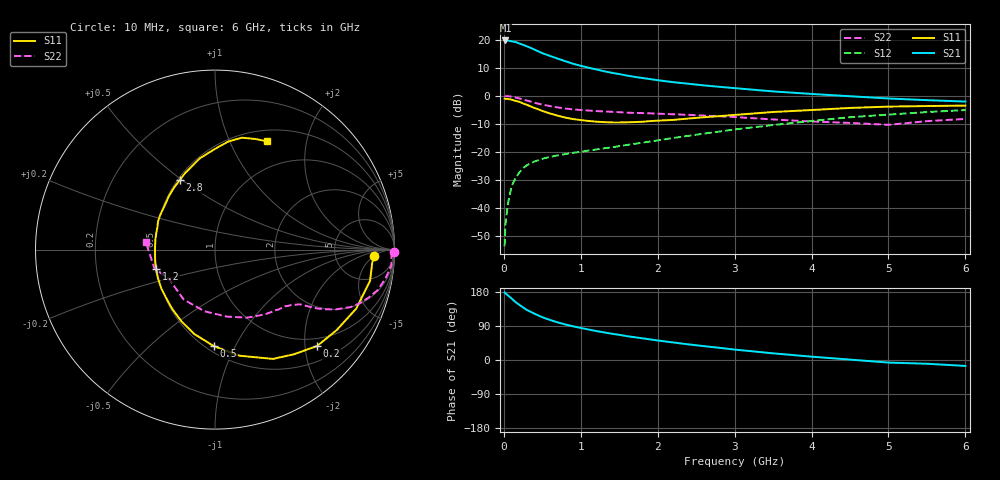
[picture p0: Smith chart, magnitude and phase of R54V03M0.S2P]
! SIEMENS Small Signal Semiconductors
! BFR183
! Si NPN RF Bipolar Junction Transistor in SOT23
! VCE = 4 V  IC = 3 mA
! Common Emitter S-Parameters:  May  1996
# GHz  S  MA  R  50
!  f  S11  S21  S12  S22
! GHz  MAG  ANG  MAG  ANG  MAG  ANG  MAG  ANG
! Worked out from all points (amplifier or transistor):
!   36 points, 10 MHz to 6 GHz, reference 50 ohm
!   highest |S21| = 19.7 dB at 20 MHz (marker M1)
!   |S21| within 3 dB of that: start of sweep to 377.3 MHz
!   unconditionally stable (mu >= 1): 1.261 GHz to 2.751 GHz
!   at 250 MHz: K = 0.29, MSG = 22.0 dB, |S12| = -25.8 dB
!   at 1.4 GHz: K = 1.05, MAG = 12.0 dB, |S12| = -18.4 dB
!   at 6 GHz: K = 0.89, MSG = 1.5 dB, |S12| = -5.1 dB
!   lowest NFmin = 1.10 dB at 450 MHz
!   S11 on the Smith chart (normalised r, x): 10 MHz: 15, -5; 200 MHz: 0.82, -2.27; 500 MHz: 0.55, -0.83; 1.2 GHz: 0.50, -0.12; 2.8 GHz: 0.51, +0.49; 6 GHz: 0.64, +1.39
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0.01  0.8886 -2.3  9.525 178.4  0.0021 91.3  0.9948 -0.9
0.02  0.8792 -4.6  9.658 176.1  0.0049 88.7  0.9839 -1.9
0.05  0.8812 -11.4  9.625 171.0  0.0115 83.1  0.9872 -5.0
0.1  0.8532 -22.6  9.326 162.5  0.0241 78.4  0.9641 -9.5
0.15  0.8128 -33.5  9.073 153.1  0.0342 71.6  0.9348 -13.9
0.2  0.7825 -43.3  8.557 145.8  0.043 67.6  0.8971 -17.3
0.25  0.7305 -53.0  8.052 138.7  0.0513 63.3  0.8609 -20.3
0.3  0.6891 -62.1  7.606 132.0  0.0581 60.2  0.8219 -22.9
0.4  0.606 -77.2  6.627 122.0  0.0677 54.7  0.7505 -26.4
0.5  0.5378 -90.7  5.735 112.9  0.0756 51.9  0.6966 -28.5
0.6  0.4848 -103.6  5.117 105.6  0.0818 49.9  0.6553 -30.0
0.7  0.4418 -114.9  4.59 99.3  0.0867 49.1  0.6209 -31.0
0.8  0.4083 -125.5  4.117 93.7  0.0918 48.9  0.5925 -31.8
1.1  0.356 -153.1  3.165 80.5  0.1058 49.8  0.5462 -34.2
1.2  0.3461 -161.7  2.945 76.5  0.1104 50.5  0.5348 -35.0
1.6  0.3372 169.8  2.288 62.9  0.133 53.5  0.501 -39.1
2.2  0.3715 139.4  1.747 46.3  0.177 55.5  0.4686 -47.8
2.8  0.4339 117.0  1.445 32.2  0.2306 53.9  0.4314 -60.0
3.5  0.5141 99.7  1.196 17.6  0.3011 48.1  0.3789 -80.1
4.5  0.6074 82.9  0.981 1.1  0.4152 36.7  0.3283 -122.1
5.5  0.6559 70.0  0.835 -9.9  0.5126 23.2  0.3534 -163.1
6  0.6693 64.2  0.789 -15.6  0.5567 14.6  0.387 174.0
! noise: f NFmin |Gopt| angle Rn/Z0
0.45  1.1  0.37  35  0.3
0.9  1.15  0.34  85  0.23
1.8  1.9  0.35  160  0.13
